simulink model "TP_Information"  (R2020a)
settings: Solver=VariableStepAuto  StartTime=0.0  StopTime=106  RelTol=1e-3
libraries: fl_lib x16, nesl_utility x3, SimscapeFluids_lib x1

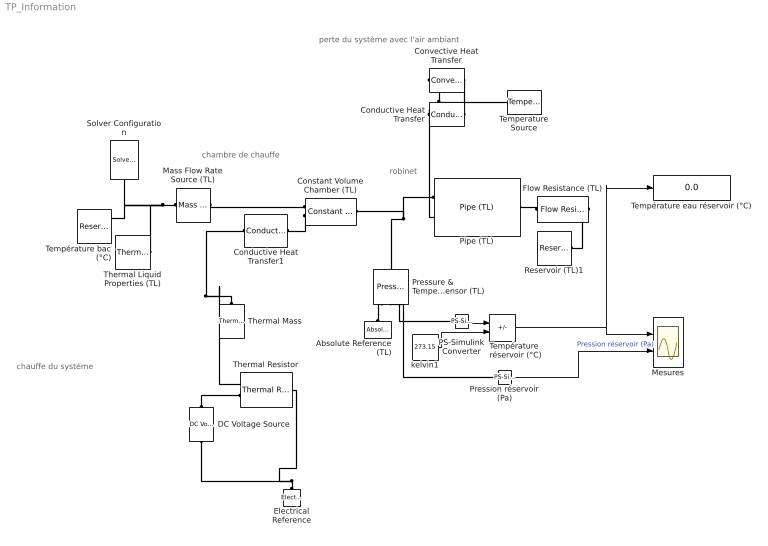
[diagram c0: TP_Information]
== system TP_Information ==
  note: robinet
  note: perte du système avec l'air ambiant
  note: chambre de chauffe
  note: chauffe du système
  Absolute Reference (TL) : fl_lib/Thermal Liquid/Elements/Absolute Reference (TL)
  Conductive Heat Transfer : fl_lib/Thermal/Thermal Elements/Conductive Heat Transfer  area=15 cm^2  thickness=0.1 cm  th_cond=2 W/(m*K)  T_specify=off  T_priority=None  T=0 K  T_nominal_specify=off  T_nominal_unit=K  T_nominal_value=1  Q_specify=off  Q_priority=None  Q=0 W  Q_nominal_specify=off  Q_nominal_unit=W  Q_nominal_value=1
  Conductive Heat Transfer1 : fl_lib/Thermal/Thermal Elements/Conductive Heat Transfer  area=30 cm^2  thickness=2 cm  th_cond=30000 W/(m*K)  T_specify=off  T_priority=None  T=0 K  T_nominal_specify=off  T_nominal_unit=K  T_nominal_value=1  Q_specify=off  Q_priority=None  Q=0 W  Q_nominal_specify=off  Q_nominal_unit=W  Q_nominal_value=1
  Constant Volume Chamber (TL) : fl_lib/Thermal Liquid/Elements/Constant Volume Chamber (TL)  volume=0.4 l  num_ports=foundation.enum.num_ports.two  area_A=0.8 cm^2  area_B=0.8 cm^2  area_C=0.01 m^2  area_D=0.01 m^2  p_I_specify=off  p_I_priority=High  p_I=0.101325 MPa  p_I_nominal_specify=off  p_I_nominal_unit=MPa  p_I_nominal_value=1  T_I_specify=off  T_I_priority=High  T_I=293.15 K  T_I_nominal_specify=off  T_I_nominal_unit=K  T_I_nominal_value=1  u_chamber_specify=off  u_chamber_priority=None  u_chamber=83.90600000000001 kJ/kg  u_chamber_nominal_specify=off  u_chamber_nominal_unit=kJ/kg  u_chamber_nominal_value=1  rho_specify=off  rho_priority=None  rho=998.21 kg/m^3  rho_nominal_specify=off  rho_nominal_unit=kg/m^3  rho_nominal_value=1
  Convective Heat Transfer : fl_lib/Thermal/Thermal Elements/Convective Heat Transfer  area=15 cm^2  heat_tr_coeff=2 W/(m^2 * K)  T_specify=off  T_priority=None  T=0 K  T_nominal_specify=off  T_nominal_unit=K  T_nominal_value=1  Q_specify=off  Q_priority=None  Q=0 W  Q_nominal_specify=off  Q_nominal_unit=W  Q_nominal_value=1
  DC Voltage Source : fl_lib/Electrical/Electrical Sources/DC Voltage Source  v0=221 V
  Electrical Reference : fl_lib/Electrical/Electrical Elements/Electrical Reference
  Flow Resistance (TL) : fl_lib/Thermal Liquid/Elements/Flow Resistance (TL)  delta_p_nominal=0.001 MPa  mdot_nominal=0.05 kg/s  area=0.4 cm^2  laminar_fraction=1e-3
  Mass Flow Rate Source (TL) : fl_lib/Thermal Liquid/Sources/Mass Flow Rate Source (TL)  commanded_mass_flow=0.033 kg/s  area=2 cm^2
  Mesures : Scope  NumInputPorts=2
  PS-Simulink Converter : nesl_utility/PS-Simulink Converter  PhysicalDomain=network_engine_domain  SubClassName=ps_output  LeftPortType=input  RightPortType=output  PseudoPeriodic=off  Frequencies=[]  Unit=inherit  AffineConversion=off
  Pipe (TL) : fl_lib/Thermal Liquid/Elements/Pipe (TL)  length=40 cm  area=2 cm^2  Dh=1 cm  length_add=1 m  roughness=15e-6 m  Re_lam=2000  Re_tur=4000  shape_factor=64  Nu_lam=3.66  dynamic_compressibility=simscape.enum.onoff.on  inertia=simscape.enum.onoff.off  p0=0.101325 MPa  T0=293.15 K  mdot0=0 kg/s
  Pression réservoir (Pa) : nesl_utility/PS-Simulink Converter  PhysicalDomain=network_engine_domain  SubClassName=ps_output  LeftPortType=input  RightPortType=output  PseudoPeriodic=off  Frequencies=[]  Unit=inherit  AffineConversion=off
  Pressure & Temperature Sensor (TL) : fl_lib/Thermal Liquid/Sensors/Pressure & Temperature Sensor (TL)
  Reservoir (TL)1 : fl_lib/Thermal Liquid/Elements/Reservoir (TL)  pressure_spec=foundation.enum.pressure_spec.atmospheric  reservoir_pressure=0.101325 MPa  reservoir_temperature=20 degC  area=0.01 m^2
  Solver Configuration : nesl_utility/Solver Configuration  PhysicalDomain=network_engine_domain  SubClassName=solver  LeftPortType=input  RightPortType=generic  Tones=[]  Harmonics=[]  SimulateNoise=off  Profile=off  UseLocalSampling=off  EnableSwitchedLinearOptims=on  FrequencyDomain=off  UseCCode=off  RelTol=0.001  AbsTol=1e-06  MinStep=1e-09  ToWorkspace=off  RevertToSquareIcSolve=off  NumHomotopyIterations=100  PhasorMode=off  PhasorModeNumHarmonics=1  DoDC=off  ResidualTolerance=1e-09  UseLocalSolver=off  LocalSolverChoice=NE_BACKWARD_EULER_ADVANCER  LocalSolverSampleTime=0.001  DoFixedCost=off  MaxNonlinIter=3  MaxModeIter=2  LinearAlgebra=auto  EquationFormulation=NE_TIME_EF  DelaysMemoryBudget=1024  AutomaticFiltering=on  FilteringTimeConstant=0.001  PartitionStorageMethod=AS_NEEDED  PartitionMemoryBudget=1024  PartitionMethod=ROBUST
  Temperature Source : fl_lib/Thermal/Thermal Sources/Temperature Source  temperature=20 degC
  Température bac (°C) : fl_lib/Thermal Liquid/Elements/Reservoir (TL)  pressure_spec=foundation.enum.pressure_spec.atmospheric  reservoir_pressure=0.101325 MPa  reservoir_temperature=21 degC  area=0.01 m^2
  Température eau réservoir (°C) : Display
  Température réservoir (°C) : Sum  Inputs=+-
  Thermal Liquid Properties (TL) : SimscapeFluids_lib/Thermal Liquid/Utilities/Thermal Liquid Properties (TL)  fluid_list=fluids.thermal_liquid.utilities.enum.thermal_liquid_fluid_list.water  concentration_param_EG=fluids.thermal_liquid.utilities.enum.thermal_liquid_concentration.volume_fraction  concentration_param_PG=fluids.thermal_liquid.utilities.enum.thermal_liquid_concentration.volume_fraction  c_mass_SW=3.5e-3  c_mass_EG=0.1  c_mass_PG=0.1  c_mass_GL=0.1  c_vol_EG=0.1  c_vol_PG=0.1  beta_const_EG=2.1791 GPa  beta_const_PG=2.1791 GPa  beta_const_GL=2.1791 GPa  p_min_EG=0.01 MPa  p_min_PG=0.01 MPa  p_min_GL=0.01 MPa  p_max_EG=50 MPa  p_max_PG=50 MPa  p_max_GL=50 MPa  p_atm=0.101325 MPa
  Thermal Mass : fl_lib/Thermal/Thermal Elements/Thermal Mass  mass=0.5 kg  sp_heat=447 J/kg/K  T_specify=off  T_priority=High  T=300 K  T_nominal_specify=off  T_nominal_unit=K  T_nominal_value=1  Q_specify=off  Q_priority=None  Q=0 W  Q_nominal_specify=off  Q_nominal_unit=W  Q_nominal_value=1
  Thermal Resistor : fl_lib/Electrical/Electrical Elements/Thermal Resistor  R0=15.24 Ohm  T0=20 degC  alpha=50e-6 1/K  tc=10 s  K_d=1e-6 W/K  T_specify=off  T_priority=High  T=300 K  T_nominal_specify=off  T_nominal_unit=K  T_nominal_value=1
  kelvin1 : Constant  Value=273.15
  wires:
  Pression réservoir (Pa)/1 -> Mesures/2  "Pression réservoir (Pa)"
  PS-Simulink Converter/1 -> Température réservoir (°C)/1
  Température réservoir (°C)/1 -> Température eau réservoir (°C)/1, Mesures/1
  kelvin1/1 -> Température réservoir (°C)/2
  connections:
  Mass Flow Rate Source (TL)/RConn1 -- Constant Volume Chamber (TL)/LConn1
  Thermal Liquid Properties (TL)/RConn1 -- Température bac (°C)/LConn1 -- Solver Configuration/RConn1 -- Mass Flow Rate Source (TL)/LConn1
  Constant Volume Chamber (TL)/LConn2 -- Conductive Heat Transfer1/RConn1
  Pipe (TL)/LConn1 -- Pressure & Temperature Sensor (TL)/LConn1 -- Constant Volume Chamber (TL)/RConn1
  Pressure & Temperature Sensor (TL)/RConn3 -- PS-Simulink Converter/LConn1
  Pression réservoir (Pa)/LConn1 -- Pressure & Temperature Sensor (TL)/RConn2
  Thermal Mass/LConn1 -- Thermal Resistor/LConn1 -- Conductive Heat Transfer1/LConn1
  Flow Resistance (TL)/RConn1 -- Reservoir (TL)1/LConn1
  Conductive Heat Transfer/RConn1 -- Pipe (TL)/LConn2 -- Convective Heat Transfer/RConn1
  Conductive Heat Transfer/LConn1 -- Temperature Source/LConn1 -- Convective Heat Transfer/LConn1
  Flow Resistance (TL)/LConn1 -- Pipe (TL)/RConn1
  DC Voltage Source/LConn1 -- Thermal Resistor/LConn2
  Electrical Reference/LConn1 -- Thermal Resistor/RConn1 -- DC Voltage Source/RConn1
  Absolute Reference (TL)/LConn1 -- Pressure & Temperature Sensor (TL)/RConn1
